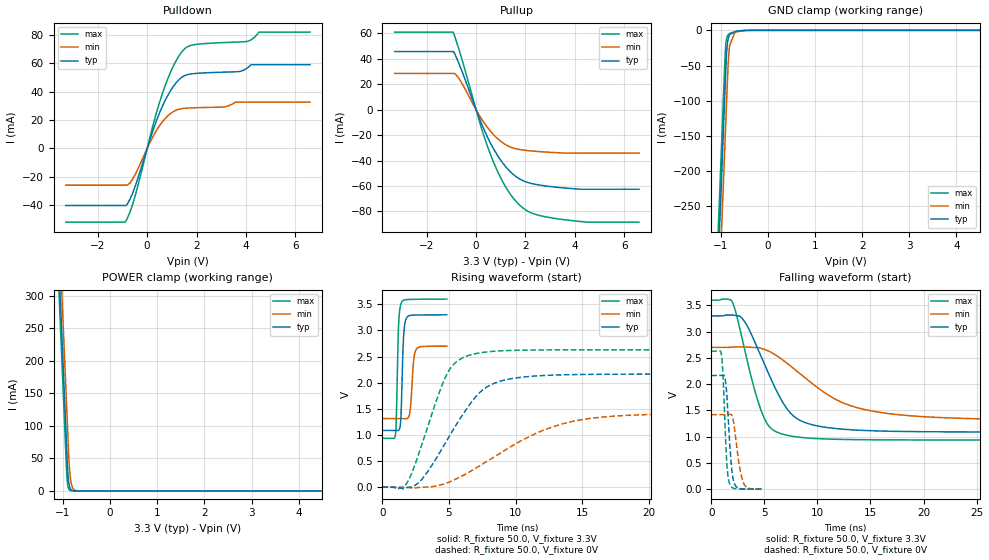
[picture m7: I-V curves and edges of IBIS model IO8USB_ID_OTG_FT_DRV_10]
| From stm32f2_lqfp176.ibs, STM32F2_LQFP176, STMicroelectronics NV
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| *** New cell (Generated with 5.14beta1 (Sep 20 2010 13:23:23))
[Model]   IO8USB_ID_OTG_FT_DRV_10
Model_type 3-state
Polarity   Non-Inverting
Enable   Active-Low
| CAP_THRESHOLD on pad IOV33 is "CMOS" :
| Rising=10.0% of vddio   Falling=90.0% of vddio
| C_comp min and max val. don't necessarily correlate with the min and max pvt
| but are the smallest and greatest pad capacitance found.
| var   typ   min   max
C_comp   2.14880pF  2.04280pF  2.27520pF
Vmeas = 1.65V   | Reference voltage for timing measurements
Cref  = 50.0pF   | Timing specification test load capacitance value
Rref  = 10.0MOhm   | Timing specification test load resistance value
Vref  = 1.65V   | Timing specification test load voltage
[Model Spec]
| variable   typ   min   max
[Temperature Range] 25.0 125.0 -40.0
| variable   typ   min   max
[Voltage Range] 3.3V 2.7V 3.6V
| variable   typ   min   max
[POWER Clamp Reference] 3.3V 2.7V 3.6V
| variable   typ   min   max
[GND Clamp Reference] 0V 0V 0V
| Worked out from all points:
|   slope of the pulldown table from 0 to 0.495 V, typ, clamps not added: 20 ohm
|   slope of the pullup table from 0 to 0.495 V, typ, clamps not added: 21.7 ohm
|   GND clamp passes 1 mA (typ) near -0.62 V on its own axis
|   POWER clamp passes 1 mA (typ) near -0.81 V on its own axis
|   rising waveform, R_fixture 50.0, V_fixture 3.3V: 20-80 % time 162ps typ, 212ps min, 146ps max; typ from 1.09 V to 3.3 V
|   falling waveform, R_fixture 50.0, V_fixture 3.3V: 20-80 % time 3.16ns typ, 6.11ns min, 2.07ns max; typ from 3.3 V to 1.09 V
|   rising waveform, R_fixture 50.0, V_fixture 0V: 20-80 % time 3.27ns typ, 6.09ns min, 2.16ns max; typ from 0 V to 2.17 V
|   falling waveform, R_fixture 50.0, V_fixture 0V: 20-80 % time 416ps typ, 602ps min, 330ps max; typ from 2.17 V to 0 V
[POWER Clamp]
-3.3V     4.11A      4.173A     4.072A
-1.09V    352.5mA    415.9mA    314.5mA
-1.05V    284.5mA    347.9mA    246.5mA
-1.01V    216.5mA    279.9mA    178.5mA
-920mV    63.51mA    126.9mA    25.85mA
-900mV    31.51mA    92.9mA     9.552mA
-890mV    21.35mA    75.9mA     5.807mA
-870mV    9.804mA    44.01mA    2.146mA
-840mV    3.05mA     18.36mA    482.1uA
-780mV    295.2uA    3.194mA    24.34uA
-660mV    2.764uA    96.54uA    62.42nA
6.6V      0A         0A         0A
[GND Clamp]
-3.3V     -4.149A    -4.223A    -4.103A
-1.06V    -340.6mA   -415.4mA   -294.6mA
-940mV    -136.6mA   -211.4mA   -90.55mA
-910mV    -85.56mA   -160.4mA   -39.55mA
-900mV    -68.56mA   -143.4mA   -26.56mA
-880mV    -36.74mA   -109.4mA   -13.48mA
-860mV    -19.55mA   -75.41mA   -8.247mA
-840mV    -11.31mA   -44.9mA    -5.968mA
-810mV    -6.021mA   -21.14mA   -4.415mA
-700mV    -1.968mA   -2.918mA   -1.891mA
-470mV    -106.7uA   -266.5uA   -47.83uA
6.6V      9.456nA    1.186uA    63.86pA
| variable   typ   min   max
[Pullup Reference] 3.3V 2.7V 3.6V
| variable   typ   min   max
[Pulldown Reference] 0V 0V 0V
[Pullup]
-3.3V     45.79mA    28.55mA    61.1mA
-930mV    45.79mA    28.55mA    61.1mA
-700mV    36.69mA    24.77mA    47.9mA
120mV     -6.142mA   -4.065mA   -8.189mA
590mV     -26.5mA    -17.07mA   -35.52mA
1.18V     -44.36mA   -27.27mA   -60.11mA
1.54V     -51.43mA   -30.39mA   -70.35mA
1.89V     -55.75mA   -31.69mA   -77.18mA
2.48V     -58.98mA   -32.83mA   -82.75mA
3.6V      -61.62mA   -34.07mA   -86.61mA
4.51V     -62.54mA   -34.07mA   -88.51mA
6.6V      -62.54mA   -34.07mA   -88.51mA
[Pulldown]
-3.3V     -40.25mA   -25.94mA   -51.99mA
-870mV    -40.25mA   -25.94mA   -51.33mA
-700mV    -35.92mA   -24.51mA   -45.06mA
-470mV    -25.89mA   -17.87mA   -32.39mA
240mV     12.97mA    8.52mA     16.62mA
590mV     28.62mA    18.11mA    37.2mA
1.07V     43.85mA    26mA       58.31mA
1.54V     51.42mA    28.24mA    70.48mA
2.01V     52.82mA    28.63mA    73.27mA
4.01V     56.01mA    32.56mA    75.18mA
4.53V     58.9mA     32.56mA    81.88mA
6.6V      58.9mA     32.56mA    81.88mA
[Ramp]
dV/dt_r 1.29886V/3.26613ns 851.30598mV/6.09251ns 1.57728V/2.15545ns
dV/dt_f 1.32782V/3.15641ns 831.60155mV/6.11557ns 1.59819V/2.06998ns
R_load = 50.0
| Removed startup time: 0s 0s 0s  .
| Removed end time: 4.838ns.
[Rising Waveform]
R_fixture   = 50.0
V_fixture   = 3.3V
V_fixture_min = 2.7V
V_fixture_max = 3.6V
0s        1.087V     1.314V     936.3mV
981ps     1.087V     1.314V     1.007V
1.043ns   1.086V     1.314V     1.292V
1.205ns   1.086V     1.314V     3.059V
1.427ns   1.576V     1.314V     3.532V
1.581ns   2.846V     1.313V     3.576V
1.801ns   3.233V     1.308V     3.589V
2.083ns   3.287V     1.468V     3.592V
2.529ns   3.294V     2.633V     3.595V
4.84ns    3.299V     2.698V     3.599V
| Removed startup time: 0s 0s 0s  .
| Removed end time: 43.595ns.
[Falling Waveform]
R_fixture   = 50.0
V_fixture   = 3.3V
V_fixture_min = 2.7V
V_fixture_max = 3.6V
0s        3.3V       2.7V       3.6V
1.94ns    3.316V     2.705V     3.58V
3.1ns     3.203V     2.71V      2.693V
4.755ns   2.496V     2.68V      1.465V
5.515ns   2.147V     2.619V     1.18V
6.7ns     1.665V     2.466V     1.049V
9.16ns    1.246V     2.068V     973.2mV
12.3ns    1.144V     1.653V     947.5mV
15.96ns   1.107V     1.46V      939.7mV
43.6ns    1.087V     1.315V     936.3mV
| Removed startup time: 0s 0s 0s  .
| Removed end time: 34.12ns.
[Rising Waveform]
R_fixture   = 50.0
V_fixture   = 0V
V_fixture_min = 0V
V_fixture_max = 0V
0s        7.764nV    280.7nV    5.722nV
1.835ns   -7.993mV   -1.583mV   78.53mV
2.99ns    159.9mV    -1.83mV    836.5mV
4.79ns    873mV      76.22mV    2.134V
6.56ns    1.583V     295.9mV    2.527V
7.67ns    1.888V     467.4mV    2.583V
9.06ns    2.043V     686.8mV    2.611V
11.91ns   2.135V     1.073V     2.626V
14.96ns   2.157V     1.291V     2.628V
34.13ns   2.165V     1.419V     2.629V
| Removed startup time: 0s 0s 0s  .
| Removed end time: 4.728ns.
[Falling Waveform]
R_fixture   = 50.0
V_fixture   = 0V
V_fixture_min = 0V
V_fixture_max = 0V
0s        2.165V     1.419V     2.629V
967ps     2.166V     1.419V     2.545V
1.142ns   2.171V     1.419V     2.016V
1.357ns   2.024V     1.418V     884.8mV
1.524ns   1.597V     1.42V      330.9mV
1.715ns   922.6mV    1.426V     107.2mV
1.984ns   285.1mV    1.384V     28.47mV
2.276ns   64.43mV    1.007V     9.737mV
3.06ns    4.925mV    107.1mV    1.686mV
4.73ns    425.6uV    740.3uV    311.6uV
